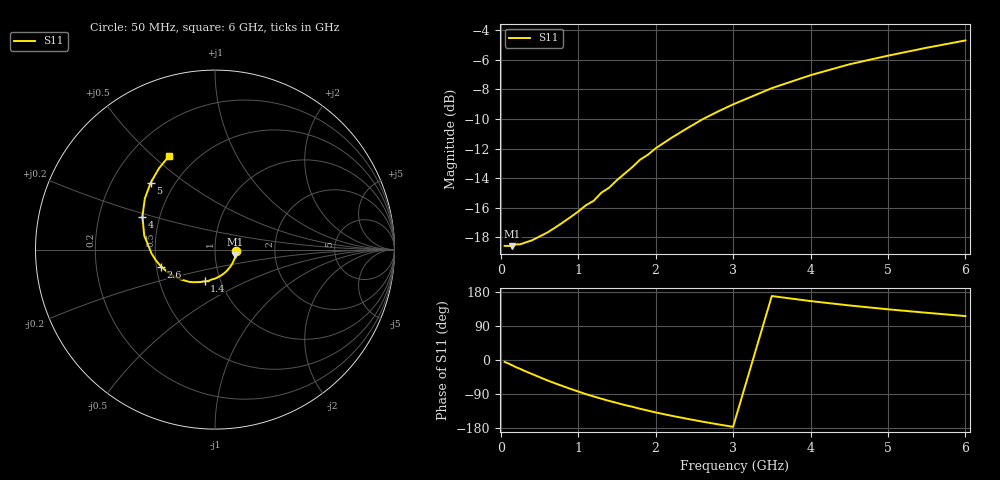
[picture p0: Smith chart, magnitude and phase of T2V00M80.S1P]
! SIEMENS Discrete & RF Semiconductors
! BAS70-04W
! Si Schottky Diode in SOT323
! IF = 0.8 mA
! S-Parameters:  November  1997
# GHz  S  MA  R  50
!  f  S11
! GHz  MAG  ANG
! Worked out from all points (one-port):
!   34 points, 50 MHz to 6 GHz, reference 50 ohm
!   lowest |S11| = -18.6 dB at 150 MHz (marker M1), VSWR 1.27, Z = 62.7 - j3.7 ohm
!   |S11| at or under -10 dB: start of sweep to 2.614 GHz
!   S11 on the Smith chart (normalised r, x): 50 MHz: 1.27, -0.03; 1.4 GHz: 0.84, -0.31; 2.6 GHz: 0.53, -0.11; 4 GHz: 0.40, +0.18; 5 GHz: 0.37, +0.38; 6 GHz: 0.36, +0.57
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0.05  0.1179 -5.1
0.15  0.1177 -14.3
0.2  0.1193 -19.2
0.25  0.1193 -23.3
0.4  0.123 -36.6
0.6  0.1307 -53.7
0.8  0.1414 -68.8
1  0.154 -83.1
1.1  0.1617 -90.1
1.2  0.1674 -96.2
1.3  0.1783 -102.2
1.4  0.1854 -108.0
1.6  0.2068 -118.8
1.7  0.2176 -123.4
1.8  0.2305 -128.8
1.9  0.2394 -133.5
2  0.2517 -138.4
2.2  0.2725 -146.9
2.4  0.2933 -154.9
2.6  0.3148 -162.5
2.8  0.3346 -169.6
3  0.3541 -176.4
3.5  0.4017 168.8
4  0.4443 155.5
4.5  0.4834 144.0
5  0.5171 133.8
5.5  0.55 124.6
6  0.582 115.9
